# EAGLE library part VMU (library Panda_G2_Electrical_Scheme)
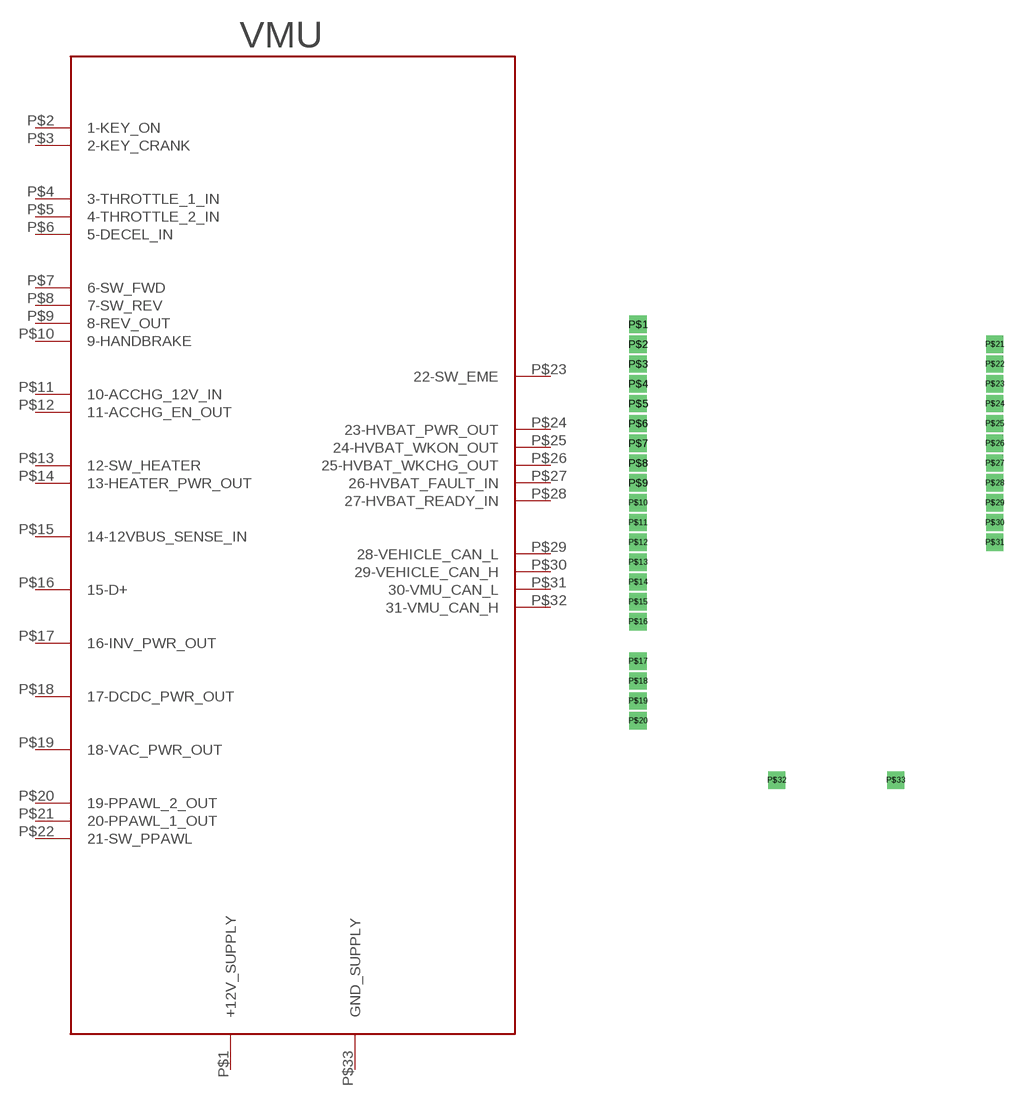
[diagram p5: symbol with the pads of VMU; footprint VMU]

Designator prefix -

## VMU  [VMU]
P$1  +12V_SUPPLY
P$2  1-KEY_ON  in
P$3  2-KEY_CRANK  in
P$4  3-THROTTLE_1_IN  in
P$5  4-THROTTLE_2_IN  in
P$6  5-DECEL_IN  in
P$7  6-SW_FWD  in
P$8  7-SW_REV  in
P$9  8-REV_OUT  out
P$10  9-HANDBRAKE  in
P$11  10-ACCHG_12V_IN  in
P$12  11-ACCHG_EN_OUT  out
P$13  12-SW_HEATER  in
P$14  13-HEATER_PWR_OUT  out
P$15  14-12VBUS_SENSE_IN  in
P$16  15-D+  out
P$17  16-INV_PWR_OUT  out
P$18  17-DCDC_PWR_OUT  out
P$19  18-VAC_PWR_OUT  out
P$20  19-PPAWL_2_OUT  out
P$21  20-PPAWL_1_OUT  out
P$22  21-SW_PPAWL  in
P$23  22-SW_EME  in
P$24  23-HVBAT_PWR_OUT  out
P$25  24-HVBAT_WKON_OUT  out
P$26  25-HVBAT_WKCHG_OUT  out
P$27  26-HVBAT_FAULT_IN  in
P$28  27-HVBAT_READY_IN  in
P$29  28-VEHICLE_CAN_L
P$30  29-VEHICLE_CAN_H
P$31  30-VMU_CAN_L
P$32  31-VMU_CAN_H
P$33  GND_SUPPLY

## Footprint VMU (pad centres in mm)
drill 0.6 square: P$1 0,31.75; P$2 0,30.48; P$3 0,29.21; P$4 0,27.94; P$5 0,26.67; P$6 0,25.4; P$7 0,24.13; P$8 0,22.86; P$9 0,21.59; P$10 0,20.32; P$11 0,19.05; P$12 0,17.78; P$13 0,16.51; P$14 0,15.24; P$15 0,13.97; P$16 0,12.7; P$17 0,10.16; P$18 0,8.89; P$19 0,7.62; P$20 0,6.35; P$21 22.86,30.48; P$22 22.86,29.21; P$23 22.86,27.94; P$24 22.86,26.67; P$25 22.86,25.4; P$26 22.86,24.13; P$27 22.86,22.86; P$28 22.86,21.59; P$29 22.86,20.32; P$30 22.86,19.05; P$31 22.86,17.78; P$32 8.89,2.54; P$33 16.51,2.54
